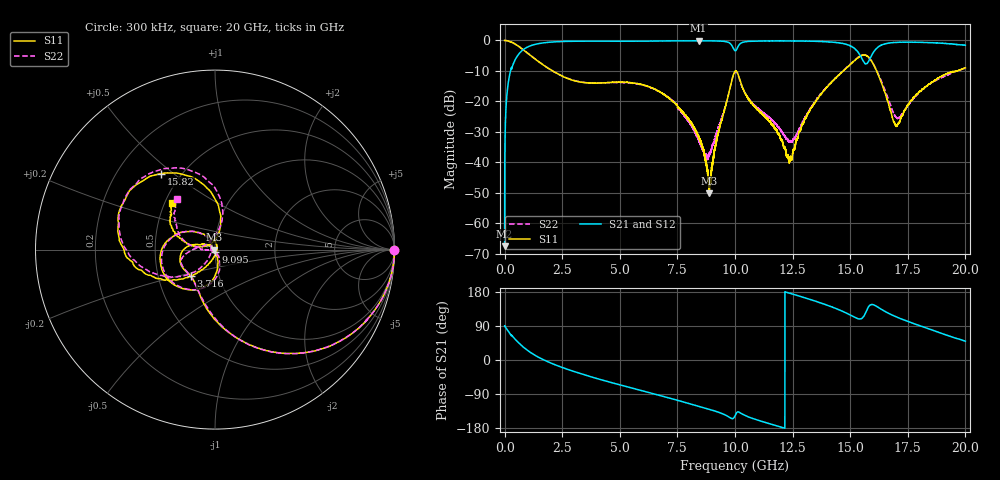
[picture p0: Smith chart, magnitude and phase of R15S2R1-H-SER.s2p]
!{R15S2R1}
!Johanson Technology Inc.
!www.johansontechnology.com
!Test Board Conditions:
!Substrate Type  RO4350B
!Substrate Thickness  20 mil
!Substrate Dk  3.66
!TL Type: GCPW
!TL Trace Width  34 mil
!TL Gap  10 mil
!Electrode orientation  Horizontal
!DUT TOPOLOGY	SERIES
!Mounting Pad LxW  26x52 mil
! Created Sat Feb  6 13:49:21 2021
# hz S ma R 50
! 2 Port Network Data from SP1.SP block
! freq  magS11  angS11  magS21  angS21  magS12  angS12  magS22  angS22
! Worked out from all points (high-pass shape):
!   20001 points, 300 kHz to 20 GHz, reference 50 ohm
!   highest |S21| = -0.10 dB at 8.417 GHz (marker M1); lowest = -67.6 dB at 300 kHz (marker M2)
!   |S21| within 3 dB of the highest: 795.4 MHz to 9.971 GHz (9.176 GHz wide, 170 % of centre); 10.06 GHz to 15.25 GHz (5.192 GHz wide, 41 % of centre)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
!   lowest |S11| = -50.2 dB at 8.888 GHz (marker M3), VSWR 1.01, Z = 49.7 - j0.0951 ohm
!   |S11| at or under -10 dB: 2.08 GHz to 10.02 GHz (7.944 GHz wide, 131 % of centre); 10.04 GHz to 14.71 GHz (4.663 GHz wide, 37.7 % of centre); 16.15 GHz to 19.67 GHz (3.518 GHz wide, 19.6 % of centre)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
!   |S22| runs from -39.1 to 0.0 dB; largest |S21 - S12| = 0.013
!   S11 on the Smith chart (normalised r, x): 300 kHz: open; 3.716 GHz: 0.73, -0.23; 9.095 GHz: 1.00, -0.03; 15.82 GHz: 0.39, +0.45; 20 GHz: 0.55, +0.33
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300000  1 -0.2  0.0004182 90.0  0.0003665 97.5  0.9979 -0.1
1.303e8  0.9852 -11.4  0.1667 78.2  0.1673 78.3  0.9847 -11.4
4.803e8  0.8627 -36.3  0.4999 53.4  0.5015 53.5  0.8617 -36.3
1.5523e9  0.428 -85.4  0.8972 4.7  0.8988 4.7  0.4288 -84.6
3.3343e9  0.2064 -126.0  0.9728 -36.6  0.9723 -36.6  0.2074 -127.0
3.7163e9  0.2003 -132.3  0.9733 -43.7  0.9726 -43.7  0.1997 -135.0
6.6673e9  0.1484 172.0  0.9783 -92.5  0.9793 -92.5  0.1484 -174.7
8.4173e9  0.02616 143.3  0.9881 -121.9  0.9855 -121.8  0.0237 -168.4
8.8883e9  0.00308 -161.9  0.9832 -130.2  0.9839 -130.2  0.01368 -97.3
9.0953e9  0.01403 -81.5  0.9822 -134.1  0.9827 -134.1  0.02167 -67.5
9.7243e9  0.1323 -87.7  0.9254 -150.0  0.9262 -149.9  0.1317 -81.5
1.00003e10  0.3105 -146.8  0.6812 -147.8  0.6823 -147.7  0.3026 -145.9
1.03043e10  0.176 144.8  0.9204 -142.3  0.9208 -142.3  0.175 144.7
1.23773e10  0.01111 -17.5  0.9813 176.2  0.9821 176.2  0.02163 172.0
1.33343e10  0.08032 -111.0  0.9724 158.3  0.9744 158.4  0.08345 -125.2
1.49653e10  0.3879 -158.2  0.8291 119.8  0.8282 119.7  0.3967 -163.5
1.54703e10  0.5566 165.5  0.5394 108.7  0.5363 108.1  0.5669 160.8
1.58183e10  0.5187 125.4  0.4696 142.3  0.4688 141.8  0.5203 119.4
1.66673e10  0.09004 77.8  0.9064 123.0  0.9012 123.4  0.1062 80.1
1.70453e10  0.04058 132.2  0.9322 112.6  0.9292 112.9  0.05279 125.6
1.80623e10  0.1471 168.5  0.9285 89.4  0.9305 89.7  0.1472 168.6
2e10  0.3542 132.4  0.8323 49.5  0.8254 49.3  0.352 126.6
